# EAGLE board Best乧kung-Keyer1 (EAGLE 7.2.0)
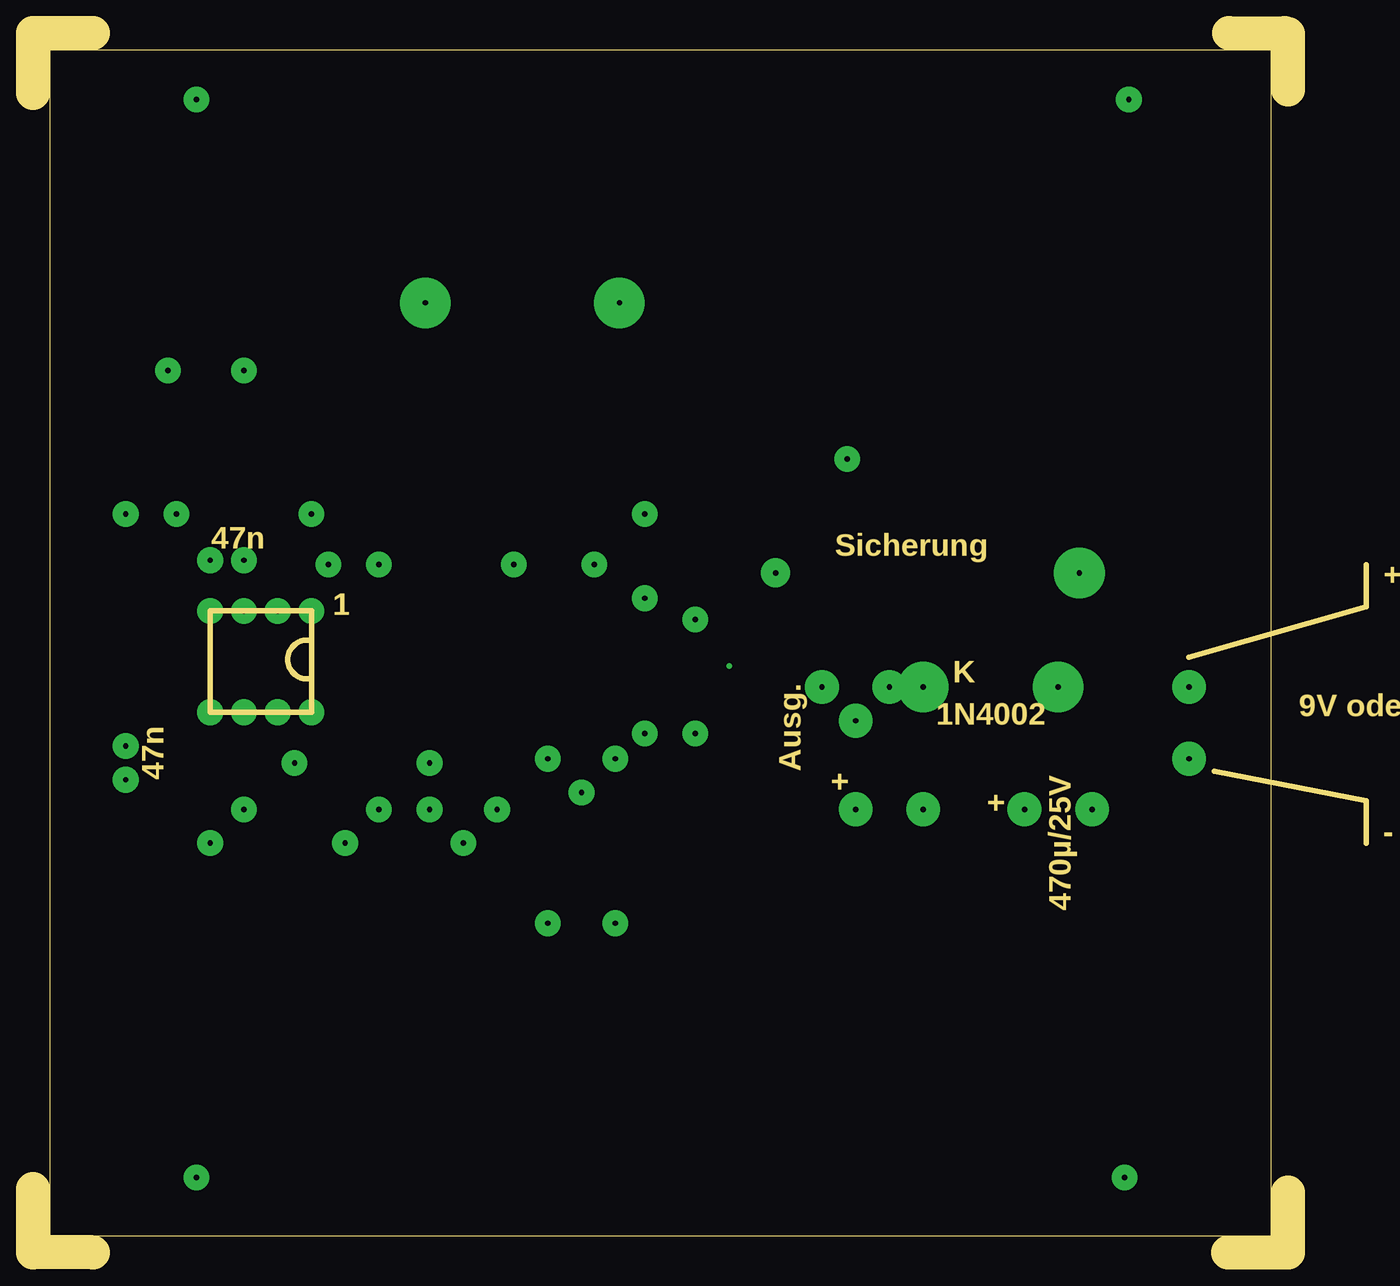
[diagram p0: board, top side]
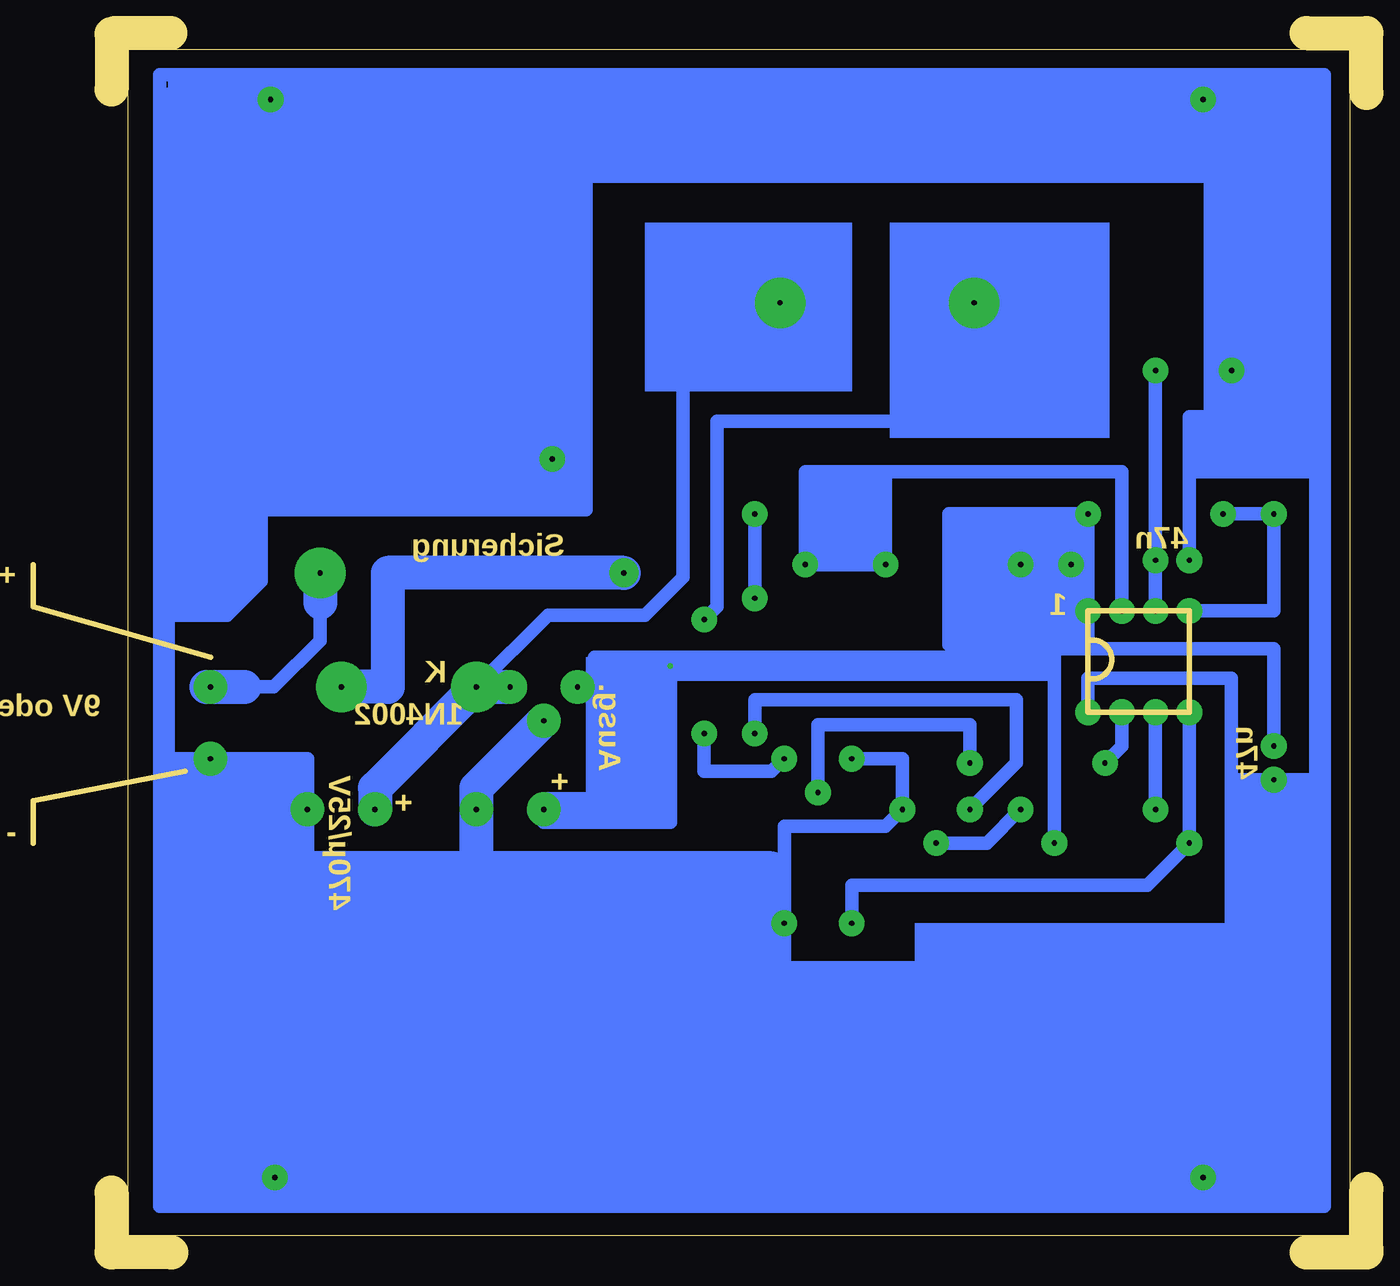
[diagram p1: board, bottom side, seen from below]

Size 100.31 x 91.7 mm. Coordinates in mm from the lower left corner, seen from the top.
Outline: 93.16,90.45 93.16,1.25 1.25,1.25 1.25,90.45
Outline: 0,87.2 0,91.7 4.5,91.7
Outline: 0,0.25 0,4.75
Outline: 4.5,0 0,0
Outline: 94.41,91.63 94.41,87.45
Outline: 94.41,4.5 94.41,0 89.91,0
Outline: 89.97,91.7 94.16,91.7
Outline: 20.93,46.02 20.93,48.24 13.31,48.24 13.31,40.62 20.93,40.62 20.93,43.16
Outline: 20.93,46.02 20.93,43.16
Outline: 20.93,43.16 arc-205 20.93,46.02
Outline: 1.25,90.47 3.16,90.47
Outline: 3.16,90.47 3.16,90.78
Outline: 3.16,90.47 93.33,90.47
Outline: 86.97,44.75 100.31,48.56 100.31,51.73
Outline: 88.88,36.17 100.31,33.95 100.31,30.78
Copper layers (1*16): Top 0.035mm / dielectric 1.5mm / Bottom 0.035mm
Design rules "default": minimum track width 10mil, minimum drill 24mil, track to track 8mil, track to pad 8mil, pad to pad 8mil, via to via 8mil, smd to smd 8mil, copper to edge 40mil, drill to drill 8mil, minimum pad ring 10mil, minimum via ring 8mil, stop-mask expansion 4mil, vias tented up to drill 0mil, thermal gap 10mil

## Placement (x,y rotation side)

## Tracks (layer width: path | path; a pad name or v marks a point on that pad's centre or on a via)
S$1  (via drill 0.4 pad 1.93)
  other vias: 12.28,5.62
S$2  (via drill 0.4 pad 1.93)
  other vias: 12.28,86.72
S$3  (via drill 0.4 pad 1.93)
  other vias: 82.12,5.62
S$4  (via drill 0.4 pad 1.93)
  other vias: 82.44,86.72
S$5
  Bottom 1.016: 58.08,44.75 23.79,44.75
S$6  (via drill 0.4 pad 2.54)
  Bottom 1.016: 52.69,42.52 v59.35,42.52
S$7  (via drill 0.4 pad 1.93)
  Bottom 1.016: v15.86,40.62 v15.86,33.32
S$8  (via drill 0.4 pad 1.93)
  other vias: 43.8,24.75
S$9  (via drill 0.4 pad 1.93)
  Bottom 1.016: v20.93,40.62 20.93,43.16 10.14,43.16 10.14,20.93
S$10
  Bottom 1.016: 11.09,61.58 11.09,81.26
S$11
  Bottom 1.016: 90.47,47.92 85.7,47.92 83.17,50.46 83.17,55.54
S$12
  Bottom 1.016: 11.73,81.26 11.73,62.21
S$13  (via drill 0.4 pad 1.93)
  Bottom 1.016: v38.72,37.13 34.91,37.13 v34.91,33.32 36.17,32.05 43.8,32.05 43.8,12.04
S$14  (via drill 0.4 pad 1.93)
  other vias: 22.2,51.73
S$17  (via drill 0.4 pad 1.93)
  other vias: 6.96,35.54
S$18  (via drill 0.4 pad 2.54, 0.4 pad 3.81)
  Bottom 1.016: v86.97,42.52 84.44,42.52 82.21,42.52 78.72,46.02 78.72,48.88
  Bottom 2.54: v78.72,51.1 78.72,48.88 | 87.29,42.52 84.44,42.52
S$19  (via drill 0.4 pad 1.93)
  other vias: 15.86,52.05
S$22  (via drill 0.4 pad 2.54)
  Bottom 1.016: 90.15,37.45 90.15,37.13 v86.97,37.13 79.67,37.13 v79.67,33.32 79.67,26.97 64.43,26.97 | 90.15,37.45 90.15,47.29 | 90.15,37.45 90.15,29.51
S$26  (via drill 0 pad 0, 0 pad 0.25, 0.4 pad 1.93, 0.4 pad 2.18, 0.4 pad 2.54, 0.4 pad 3.81)
  Bottom 1.016: v43.8,37.13 44.75,36.17 49.83,36.17 v49.83,39.03 | v49.83,47.6 48.88,48.56 48.88,62.53 29.51,62.53 v29.51,71.42 | 73.64,42.52 v77.13,42.52 | v15.86,48.24 v15.86,66.34 | v18.39,48.24 18.39,58.72 36.17,58.72 | v20.93,48.24 20.93,45.38 19.66,45.38 | 19.66,45.38 6.96,45.38 6.96,42.84 | 6.96,42.84 6.96,43.16 | v6.96,38.08 6.96,42.84 | 23.48,43.48 v23.48,30.78 | 23.48,43.48 23.48,45.38 19.66,45.38 | 23.48,43.48 53,43.48 | 10.14,35.54 3.79,35.54 3.79,58.72 | 3.79,62.84 3.79,64.43 3.16,64.43 3.16,63.48 | 3.79,62.84 3.79,58.72 | 14.9,11.73 90.78,11.73 | 14.9,11.73 13.63,11.73 | 3.16,12.68 3.16,12.36 | 3.16,12.68 3.16,63.48 | 3.16,11.73 3.16,12.68 | 3.16,11.73 14.9,11.73 | v13.31,52.05 13.31,62.84 3.79,62.84 | v13.31,48.24 6.96,48.24 v6.96,55.54 v10.78,55.54 | v20.93,48.24 v20.93,55.54 | v20.93,55.54 v26.02,51.73 | 36.17,58.72 v36.17,51.73 v42.21,51.73 42.21,58.72 36.17,58.72 | v46.02,49.19 v46.02,55.54 | 61.89,32.36 52.37,32.36 v52.37,44.11 | 90.78,55.23 90.78,56.18 | 90.78,55.23 90.78,58.4 | 90.78,58.4 90.78,59.67 v61.26,59.67 | 26.02,48.24 v26.02,51.73 | v26.02,51.73 26.02,55.54 25.7,55.54 | v20.93,55.54 25.7,55.54 | v20.93,48.24 26.02,48.24 | 26.02,48.24 26.02,44.75 | 25.7,55.54 31.41,55.54 31.41,45.7 | 3.79,58.72 13,58.72 | v61.26,59.67 61.26,55.86 61.89,55.86 | 61.89,55.86 84.75,55.86 | v44.11,71.42 51.41,71.42 51.41,50.78 54.27,47.92 61.58,47.92 v66.97,42.52 v64.43,42.52 | 3.16,11.73 3.16,3.47 90.78,3.47 90.78,55.23 | 3.16,63.48 3.16,88.56 16.81,88.56 | 16.81,88.56 90.78,88.56 90.78,58.4 | v61.26,59.67 61.26,88.25 | 61.89,55.86 58.72,55.86 58.72,88.25 | 16.81,88.56 16.81,80.94 16.17,80.94 | 16.17,80.94 10.14,80.94 v10.14,66.34 10.14,61.26
  Bottom 1.016: 16.17,80.94 61.58,80.94
  Bottom 2.184: 24.11,44.11 v52.37,44.11
  Bottom 2.54: v55.86,51.1 73.64,51.1 73.64,42.52 77.45,42.52 | v64.43,42.52 v66.97,42.52 74.59,34.91 v74.59,33.32
S$27
  Bottom 2.54: 44.75,28.87 89.52,28.87
S$28  (via drill 0.4 pad 1.93)
  Bottom 1.016: v13.31,40.62 v13.31,30.78 16.49,27.6 21.25,27.6 | v38.72,24.75 38.72,27.6 37.45,27.6 | 37.45,27.6 38.08,27.6 | 21.25,27.6 20.3,27.6 | 21.25,27.6 37.45,27.6
S$29  (via drill 0.4 pad 1.93)
  Bottom 1.016: v26.02,33.32 28.55,30.78 v32.36,30.78
S$32  (via drill 0.4 pad 2.54)
  Bottom 2.54: v61.89,39.98 66.97,34.91 66.97,29.51
S$33  (via drill 0.4 pad 2.54)
  other vias: 66.97,33.32
S$35  (via drill 0.4 pad 1.93)
  Bottom 1.016: v18.39,40.62 18.39,38.08 v19.66,36.81
S$36  (via drill 0.4 pad 1.93)
  Bottom 1.016: v29.82,33.32 26.33,36.81 26.33,41.57 41.26,41.57 | 41.26,41.57 41.89,41.57 | v46.02,39.03 46.02,41.57 41.26,41.57
S$38  (via drill 0.4 pad 1.93)
  Bottom 1.016: v41.26,34.59 41.26,39.67 29.82,39.67 v29.82,36.81
S$39  (via drill 0.4 pad 2.54)
  Bottom 2.54: 53.64,33.32 v61.89,33.32
S$91
  Bottom 1.016: 38.72,44.11 52.69,44.75
  Bottom 2.184: 38.72,44.11 53.32,44.11
(copper drawn outside any net)
  shapes: Bottom area x28

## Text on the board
Vias: Auf Bestückungsseite gesehen !
Dimension: BEI ANDEREM SUMMER MÜSSEN | DIE LÖCHER GEÄNDERT WERDEN ! | 88,9mm | 47n | Sicherung | + | 1 | K | 9V oder 12V | 1N4002 | Ausg. | 47n | + | + | - | 470µ/25V | K | Cevausit 1,5mm dick | alles mit 0,8mm vorgebohrt | Aufbohren wie folgt: | HIER AUFTRENNEN BEI 5Volt-SUMMER | Summer 1,0mm | HIER BRÜCKE BEI 5Volt-SUMMER | 92,0mm
tOrigins: Die 4 Befestigungs-Bohrungen sind | Achtung : | für das angegebene Gehäuse in der Stückliste. | Der Summer ist gegen +12Volt geschaltet. | Bei neuem Summer (2019 siehe Stck-Liste) | Die Gehäusezeichnung findet man unter "Datenblatt" ! | muss er gegen +5Volt geschaltet sein. | Die Hinweise unter "Fotos" als txt-Datei auch durchlesen ! | 78L05 | Summer | Ausg. | Eing. | Poti | Poti | - | + | Masse | BC547c | Pkt. | 10K | Poti | 10K | µA78L05 | PIC12F683 oder PIC12F675 | Drossel | E | Brücke | 18K | C | E | 18K | E | BC547c | 10K | B | BC547c | 100µ/63V | 1N4002 | Str. | Masse | Katode | Anode | Diode 1N4002 1,0mm | Sicherungshalter 1,5mm | 4Stck. Befestigungsbohr... 3,2mm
